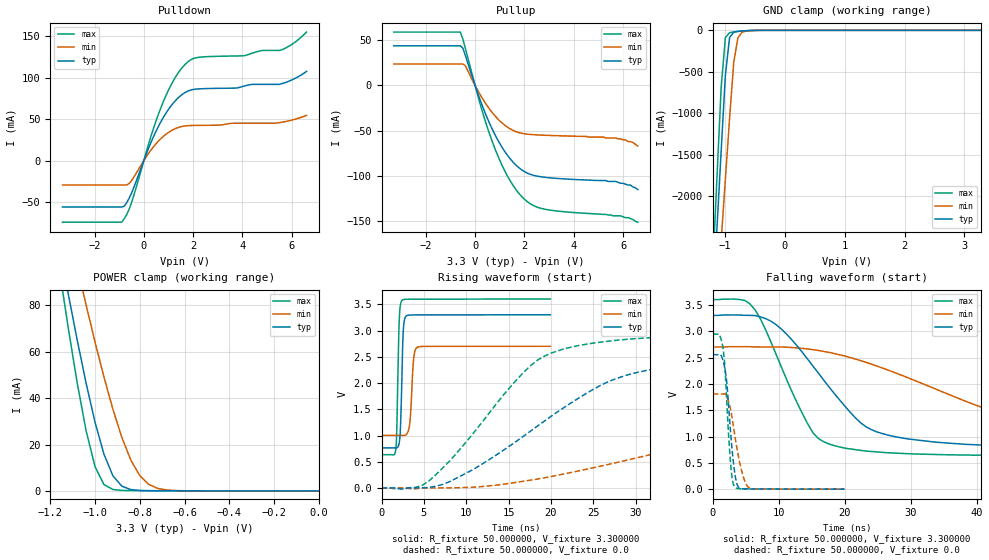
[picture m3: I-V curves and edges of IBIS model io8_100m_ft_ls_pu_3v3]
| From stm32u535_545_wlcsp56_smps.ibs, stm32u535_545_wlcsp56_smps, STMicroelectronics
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|   Model io8_100m_ft_ls_pu_3v3
[Model]  io8_100m_ft_ls_pu_3v3
Model_type I/O
Polarity   Non-Inverting
Enable   Active-Low
Vinl =   0.990000V
Vinh =   2.310000V
Vmeas =  1.650000V
Cref =   50.000000pF
Rref =   100.000000M
Vref =   0.0V
C_comp   3.313100pF   3.281800pF   3.354500pF
[Temperature Range]   25.000000   0.140000k   -40.000000
[Pullup Reference]   3.300000V   2.700000V   3.600000V
[Pulldown Reference]   0.0V   0.0V   0.0V
[POWER Clamp Reference]   3.300000V   2.700000V   3.600000V
[GND Clamp Reference]   0.0V   0.0V   0.0V
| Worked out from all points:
|   slope of the pulldown table from 0 to 0.495 V, typ, clamps not added: 14 ohm
|   slope of the pullup table from 0 to 0.495 V, typ, clamps not added: 13.7 ohm
|   GND clamp passes 1 mA (typ) near -0.51 V on its own axis
|   POWER clamp passes 1 mA (typ) near -0.85 V on its own axis
|   rising waveform, R_fixture 50.000000, V_fixture 3.300000: 20-80 % time 250ps typ, 341ps min, 234ps max; typ from 0.765 V to 3.3 V
|   rising waveform, R_fixture 50.000000, V_fixture 0.0: 20-80 % time 14.6ns typ, 31.3ns min, 9.34ns max; typ from 0.001 V to 2.55 V
|   falling waveform, R_fixture 50.000000, V_fixture 3.300000: 20-80 % time 10ns typ, 23.1ns min, 6.36ns max; typ from 3.3 V to 0.765 V
|   falling waveform, R_fixture 50.000000, V_fixture 0.0: 20-80 % time 1.02ns typ, 1.54ns min, 819ps max; typ from 2.55 V to 0.001 V
[Pulldown]
|Voltage   I(typ)   I(min)   I(max)
-3.3V     -56.06mA   -29.42mA   -74.35mA
-900mV    -56.06mA   -29.42mA   -74.35mA
-700mV    -51.09mA   -29.42mA   -65.48mA
-500mV    -39.32mA   -24.2mA    -50.88mA
300mV     22.62mA    13.13mA    30.42mA
800mV     52.54mA    29.36mA    71.75mA
1.3V      72.91mA    38.82mA    101.4mA
1.8V      84.02mA    42.13mA    119.4mA
2.3V      86.61mA    42.5mA     124.8mA
5.5V      91.97mA    45.76mA    132.8mA
6V        97.2mA     48.8mA     140mA
6.6V      107.6mA    54.5mA     155mA
[Pullup]
|Voltage   I(typ)   I(min)   I(max)
-3.3V     43.79mA    23.73mA    58.94mA
-600mV    43.79mA    23.73mA    58.94mA
-500mV    41.28mA    23.73mA    51.52mA
-400mV    33.57mA    21.9mA     41.51mA
300mV     -22.93mA   -14.5mA    -29.27mA
800mV     -54.04mA   -33.36mA   -69.41mA
1.4V      -80.24mA   -47.59mA   -104.2mA
1.7V      -89.03mA   -51.43mA   -116.5mA
2.1V      -96.56mA   -53.74mA   -127.9mA
3V        -101.9mA   -55.18mA   -137.5mA
5.7V      -106mA     -58mA      -144mA
6.6V      -115mA     -67mA      -151mA
[GND_clamp]
|Voltage   I(typ)   I(min)   I(max)
-3.3V     -9.848A    -9.957A    -9.458A
-1.2V     -3.312A    -4.013A    -2.863A
-1.13V    -2.381A    -3.274A    -1.769A
-1.06V    -1.452A    -2.535A    -684.7mA
-990mV    -542.9mA   -1.798A    -88.02mA
-920mV    -87.11mA   -1.064A    -28.44mA
-850mV    -22.1mA    -382.4mA   -19.61mA
-780mV    -11.97mA   -86.98mA   -13.71mA
-710mV    -7.619mA   -22.26mA   -8.745mA
-640mV    -4.493mA   -7.773mA   -4.817mA
-360mV    -31.22uA   -172.6uA   -8.607uA
3.28V     0A         15.66nA    -5.841nA
[POWER_clamp]
|Voltage   I(typ)   I(min)   I(max)
-3.28V    1.355A     1.167A     1.665A
-1.16V    105.8mA    131.6mA    95.87mA
-1.12V    85.08mA    114mA      70.45mA
-1.08V    65.19mA    96.88mA    46.75mA
-1.04V    46.48mA    80.2mA     25.96mA
-1V       29.64mA    64.18mA    10.49mA
-960mV    15.81mA    49.06mA    2.743mA
-920mV    6.481mA    35.16mA    612.9uA
-840mV    578.2uA    13.29mA    138.5uA
-760mV    94.37uA    2.807mA    98.56uA
-640mV    40.55uA    159.2uA    59.96uA
0V        0A         19.29nA    0A
[Ramp]
| variable   typ   min   max
dV/dt_r  1.53214/14.61944n   1.08405/31.19692n   1.76630/9.32421n
dV/dt_f  1.52096/10.00888n   1.01838/23.04248n   1.77907/6.34892n
R_load = 50.000000
[Rising Waveform]
R_fixture= 50.000000
V_fixture= 3.300000
V_fixture_min= 2.700000
V_fixture_max= 3.600000
|time   V(typ)   V(min)   V(max)
0s        765.1mV    1.003V     634.9mV
1.682ns   763.2mV    1.003V     732.8mV
2.082ns   854.2mV    1.003V     3.17V
2.242ns   1.172V     1.002V     3.5V
2.442ns   2.35V      1.002V     3.579V
2.763ns   3.237V     1.003V     3.595V
3.323ns   3.295V     1.219V     3.597V
3.804ns   3.298V     2.477V     3.598V
4.204ns   3.298V     2.679V     3.598V
19.94ns   3.3V       2.7V       3.6V
[Rising Waveform]
R_fixture= 50.000000
V_fixture= 0.0
V_fixture_min= 0.0
V_fixture_max= 0.0
|time   V(typ)   V(min)   V(max)
0s        826.3uV    846.9uV    871.5uV
5.606ns   10.93mV    2.432mV    134.6mV
11.21ns   390.6mV    17.81mV    1.118V
16.02ns   900.3mV    110mV      2.072V
19.22ns   1.274V     193.5mV    2.512V
27.23ns   2.055V     465.3mV    2.806V
34.43ns   2.325V     740.4mV    2.884V
57.66ns   2.518V     1.489V     2.939V
86.49ns   2.55V      1.73V      2.945V
398.8ns   2.554V     1.808V     2.945V
[Falling Waveform]
R_fixture= 50.000000
V_fixture= 3.300000
V_fixture_min= 2.700000
V_fixture_max= 3.600000
|time   V(typ)   V(min)   V(max)
0s        3.3V       2.7V       3.6V
4.805ns   3.302V     2.706V     3.587V
6.406ns   3.297V     2.703V     3.405V
10.41ns   3.039V     2.7V       2.313V
16.02ns   2.203V     2.634V     960.6mV
22.42ns   1.259V     2.44V      736.7mV
26.43ns   1.031V     2.268V     692.6mV
45.65ns   814.2mV    1.384V     641.3mV
76.08ns   771.9mV    1.089V     635.4mV
398.8ns   765.1mV    1.003V     634.9mV
[Falling Waveform]
R_fixture= 50.000000
V_fixture= 0.0
V_fixture_min= 0.0
V_fixture_max= 0.0
|time   V(typ)   V(min)   V(max)
0s        2.554V     1.808V     2.945V
920.9ps   2.554V     1.808V     2.944V
1.562ns   2.438V     1.808V     2.66V
1.842ns   2.279V     1.811V     2.314V
2.082ns   2.072V     1.763V     1.754V
2.683ns   1.102V     1.521V     513.7mV
3.323ns   312mV      1.033V     41.98mV
4.525ns   7.985mV    277.4mV    7.193mV
5.606ns   4.756mV    17.89mV    6.793mV
19.94ns   826.3uV    846.9uV    871.5uV
